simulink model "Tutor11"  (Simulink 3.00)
settings: Solver=ode45  SolverMode=SingleTasking  StartTime=0.0  StopTime=10  RelTol=1e-3  AbsTol=1e-3
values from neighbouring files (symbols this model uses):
  Au = [a0 a1;a2]    [data_id1.m]    (also in data_id2.m = [a0;[a1 a2]])
  Ay = [A0 A1;A2]    [data_id1.m]    (also in data_id2.m = A0)
  Bu = [b0;b1]    [data_id1.m]    (also in data_id2.m)
  By = [B0;B1]    [data_id1.m]    (also in data_id2.m)
  Cu = [c0 c1]/den(1)    [data_id1.m]    (also in data_id2.m = [c0 c1])
  Cy = [C0;C1]/den(1)    [data_id1.m]    (also in data_id2.m = [C0;C1])
  Du = zeros(in*(cit+1),in)    [data_id1.m]    (also in data_id2.m = zeros(cit*in,in))
  Dy = -[zeros(out,out);By]/den(1)    [data_id1.m]    (also in data_id2.m = [D1;D2])
libraries: simulink3 x1

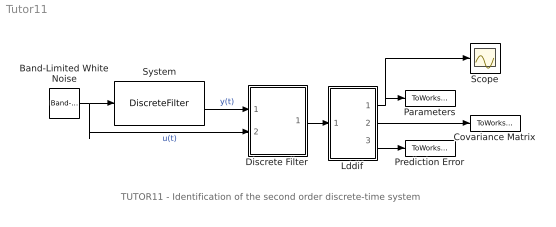
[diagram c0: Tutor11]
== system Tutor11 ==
  note: TUTOR11 - Identification of the second order discrete-time system
  Band-Limited White Noise : simulink3/Sources/Band-Limited White Noise  Cov=[0.1]  Ts=0.1  seed=[23341]
  Covariance Matrix : ToWorkspace  VariableName=CovMatrix  SampleTime=0  SaveFormat=Matrix
  Discrete Filter : Subsystem  mask(D-Filter){par=[1,1], cit=[2], men=[2], ts=[1], Ds=[0]}
      mask prompts: par "No. of inputs and outputs -  [in,out]:"; cit "Numerator degree -  [dn]:"; men "Denominator degree -  [dd]:"; ts "Sampling time - [ts]:"; Ds "Discrete time delay - [D]:"
      mask help: D-filter: Discrete filter Authors: Lubos Cirka and Miroslav Fikar 1998 - 2004
      mask init:
      | in=par(1); out=par(2);  eval('data_id2');
  Lddif : Subsystem  mask(LDDIF){par=[4,1], L=[0.985], d=[0.01], poc=[0 0 0 0], kov=[10e6], ts=[1]}
      mask prompts: par "No. of estimated parameters and outputs - [n,m]:"; L "Exponential forgetting - [L]:"; d "Bittanti's correction - [d]:"; poc "Initial parameter estimates - [theta(1) ... theta(n)]:"; kov "Covariance matrix (see help, standard - [10e6]):"; ts "Sampling period - [ts]:"
      mask help: LDDIF: + Bittanti's corrections Authors: Lubos Cirka and Miroslav Fikar 1998 - 2004
      mask init:
      | n=par(1); m=par(2);
  Parameters : ToWorkspace  VariableName=BA  SampleTime=0  SaveFormat=Matrix
  Prediction Error : ToWorkspace  VariableName=PredError  SampleTime=0  SaveFormat=Matrix
  Scope : Scope
  System : DiscreteFilter  Numerator=[0 0.8 0.2]  Denominator=[1 -0.5 0.06]  SampleTime=1
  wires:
  System/1 -> Discrete Filter/1(y)  "y(t)"
  Band-Limited White Noise/1 -> System/1, Discrete Filter/2(u)  "u(t)"
  Discrete Filter/1("y, z") -> Lddif/1("y, z")
  Lddif/2(covariance matrix) -> Covariance Matrix/1
  Lddif/3(prediction error) -> Prediction Error/1
  Lddif/1(theta) -> Parameters/1, Scope/1

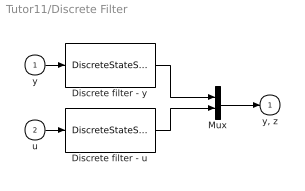
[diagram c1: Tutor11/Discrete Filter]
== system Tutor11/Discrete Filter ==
  y : Inport  Port=1  PortWidth=-1  SampleTime=-1  DataType=auto
  u : Inport  Port=2  PortWidth=-1  SampleTime=-1  DataType=auto
  Discrete filter - u : DiscreteStateSpace  A=Au  B=Bu  C=Cu  D=Du  X0=0  SampleTime=ts
  Discrete filter - y : DiscreteStateSpace  A=Ay  B=By  C=Cy  D=Dy  X0=0  SampleTime=ts
  Mux : Mux  Inputs=2
  "y, z" : Outport  Port=1  InitialOutput=0
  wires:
  y/1 -> Discrete filter - y/1
  u/1 -> Discrete filter - u/1
  Discrete filter - y/1 -> Mux/1
  Discrete filter - u/1 -> Mux/2
  Mux/1 -> "y, z"/1

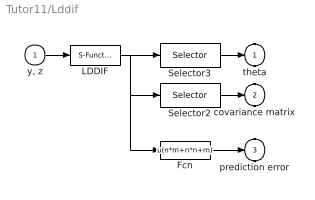
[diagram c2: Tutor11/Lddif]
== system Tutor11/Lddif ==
  "y, z" : Inport  Port=1  PortWidth=-1  SampleTime=-1  DataType=auto
  Fcn : Fcn  Expr=u(n*m+n*n+m)
  LDDIF : S-Function  FunctionName=lddif_s  Parameters=m, n, L, d, poc, kov, ts  PortCounts=[]  SFunctionModules=''
  Selector2 : Selector  Elements=[n*m:1:n*m+n*n]  InputPortWidth=n*m+n*n+m
  Selector3 : Selector  Elements=[1:1:n*m]  InputPortWidth=n*m+n*n+m
  theta : Outport  Port=1  InitialOutput=0
  covariance matrix : Outport  Port=2  InitialOutput=0
  prediction error : Outport  Port=3  InitialOutput=0
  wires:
  "y, z"/1 -> LDDIF/1
  LDDIF/1 -> Selector3/1, Selector2/1, Fcn/1
  Selector2/1 -> covariance matrix/1
  Selector3/1 -> theta/1
  Fcn/1 -> prediction error/1
